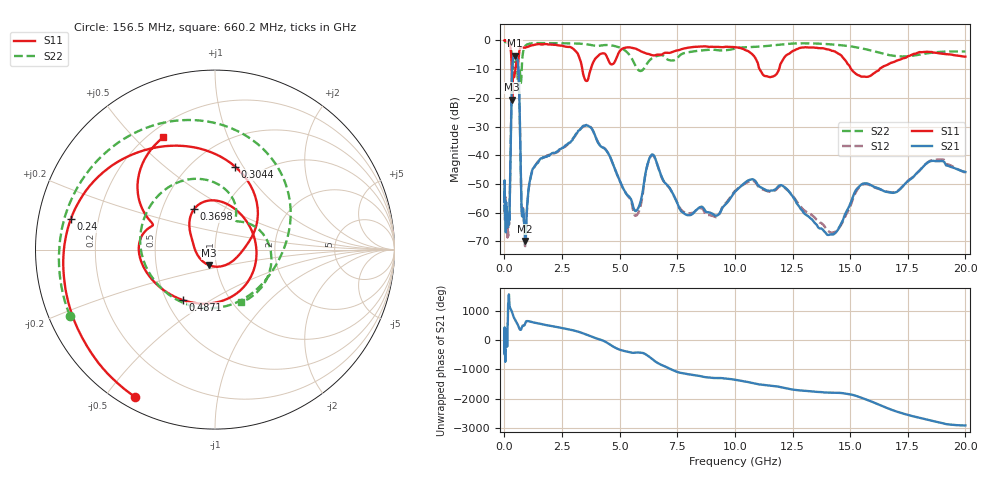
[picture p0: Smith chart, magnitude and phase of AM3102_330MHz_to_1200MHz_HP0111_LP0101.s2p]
! Date/Time: Tue, Sep 11, 2018 5:16 PM
! Network Analyzer: Agilent Technologies E8362B Rev: A.07.50.63
! Sweep from 0.010 to 20.000 GHz, 1601 Points, Sweep Type: LOG
! Power Supply: 4.949 V, 0.001 A
# Hz S DB R 50
!freq MagS11 AngS11 MagS21 AngS21 MagS12 AngS12 MagS22 AngS22
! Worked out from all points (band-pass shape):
!   1601 points, 10 MHz to 20 GHz, reference 50 ohm
!   highest |S21| = -5.23 dB at 445.1 MHz (marker M1); lowest = -69.9 dB at 899.1 MHz (marker M2)
!   |S21| within 3 dB of the highest: 350.7 MHz to 593.2 MHz (242.6 MHz wide, 51.4 % of centre)
!   lowest |S11| = -20.6 dB at 341.1 MHz (marker M3), VSWR 1.21, Z = 46.2 - j8.15 ohm
!   |S11| at or under -10 dB: 3.379 GHz to 3.748 GHz (368.9 MHz wide, 10.4 % of centre); 11.07 GHz to 11.92 GHz (846.2 MHz wide, 7.36 % of centre); 15.04 GHz to 16.28 GHz (1.234 GHz wide, 7.88 % of centre)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
!   |S22| runs from -14.8 to -0.2 dB; largest |S21 - S12| = 0.01
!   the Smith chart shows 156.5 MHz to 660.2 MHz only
!   S11 on the Smith chart (normalised r, x): 156.5 MHz: 0.05, -0.59; 240 MHz: 0.10, +0.10; 304.4 MHz: 0.77, +0.92; 369.8 MHz: 0.72, +0.35; 487.1 MHz: 0.60, -0.38; 660.2 MHz: 0.26, +0.61
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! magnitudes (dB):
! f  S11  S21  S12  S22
! 10 MHz  0.0  -49.4  -51.9  -0.2
! 35.55 MHz  0.0  -58.0  -62.4  -0.4
! 126.4 MHz  -0.4  -63.0  -62.6  -0.9
! 156.5 MHz  -0.6  -63.9  -68.3  -1.0
! 240 MHz  -1.7  -52.5  -52.9  -1.7
! 304.4 MHz  -6.5  -21.1  -21.1  -4.0
! 341.1 MHz  -20.6  -9.6  -9.7  -8.3
! 369.8 MHz  -11.9  -6.8  -6.8  -10.0
! 445.1 MHz  -11.9  -5.2  -5.3  -7.8
! 447.2 MHz  -11.8  -5.2  -5.3  -7.8
! 487.1 MHz  -9.5  -5.4  -5.5  -7.2
! 660.2 MHz  -3.2  -23.7  -23.7  -9.7
! 750.6 MHz  -2.4  -59.6  -59.2  -10.3
! 899.1 MHz  -2.5  -69.9  -71.6  -2.0
! 1.59 GHz  -1.4  -41.1  -41.2  -0.9
! 3.651 GHz  -12.9  -29.8  -29.5  -1.4
! 5.652 GHz  -2.7  -59.3  -60.9  -8.2
! 6.426 GHz  -5.1  -39.7  -40.0  -6.1
! 7.882 GHz  -2.7  -60.8  -60.2  -4.2
! 10.73 GHz  -4.6  -48.4  -48.9  -2.3
! 14.07 GHz  -3.2  -67.8  -66.6  -1.3
! 20 GHz  -5.6  -45.9  -46.1  -3.8
